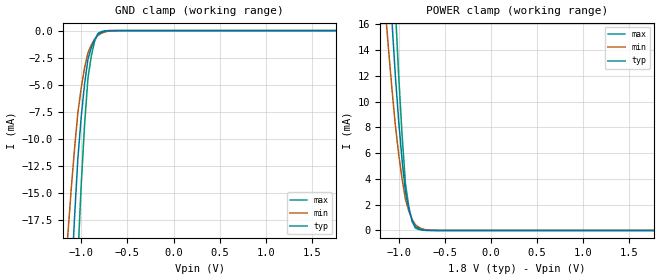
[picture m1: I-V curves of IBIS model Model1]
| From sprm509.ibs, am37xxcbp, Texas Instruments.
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| Model based on original model for IOSCHF18HYQS_SSBHV
|   Sub model IOSCHF18HYQS_SSBHV
[model]   Model1
|[Input Load]
|[Output Drive]
|Voltage   1.8V
|Mode   INPUT
Model_type   Input
Polarity   Non-Inverting
Vinl =  0.63
Vinh =  1.17
C_comp   1.157p   1.001p   1.301p
[Model Spec]
Vinl   0.63   0.567   0.6615
Vinh   1.17   1.053   1.2285
[Temperature Range]   25   125   -40
[Voltage Range]   1.8   1.62   1.89
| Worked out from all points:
|   GND clamp passes 1 mA (typ) near -0.86 V on its own axis
|   POWER clamp passes 1 mA (typ) near -0.86 V on its own axis
[POWER_clamp]
-1.8V     125.1mA    90.63mA    173.4mA
-1.145V   25.33mA    17.15mA    36.56mA
-1.109V   20.65mA    13.94mA    29.86mA
-1.073V   16.2mA     10.94mA    23.42mA
-1.036V   11.97mA    8.145mA    17.24mA
-1V       8.45mA     5.899mA    11.94mA
-963.6mV  5.452mA    3.992mA    7.408mA
-927.3mV  2.975mA    2.424mA    3.634mA
-854.5mV  779.1uA    853.1uA    686.6uA
-818.2mV  292.8uA    424.3uA    183.6uA
-600mV    1.304uA    7.605uA    175.4nA
1.764V    -20.05pA   -586.2pA   -149.6pA
[GND_clamp]
-1.8V     -189.8mA   -126.1mA   -302.4mA
-1.145V   -30.27mA   -18.93mA   -52.04mA
-1.109V   -23.46mA   -14.72mA   -40.7mA
-1.073V   -17.31mA   -10.94mA   -30.35mA
-1.036V   -11.81mA   -7.596mA   -20.99mA
-1V       -7.972mA   -5.278mA   -14.21mA
-963.6mV  -4.92mA    -3.43mA    -8.677mA
-927.3mV  -2.657mA   -2.051mA   -4.393mA
-854.5mV  -808.7uA   -794.4uA   -965uA
-818.2mV  -350.6uA   -438.9uA   -248.4uA
-600mV    -612.5nA   -5.16uA    -65.45nA
1.764V    15.58pA    1.6nA      229pA
